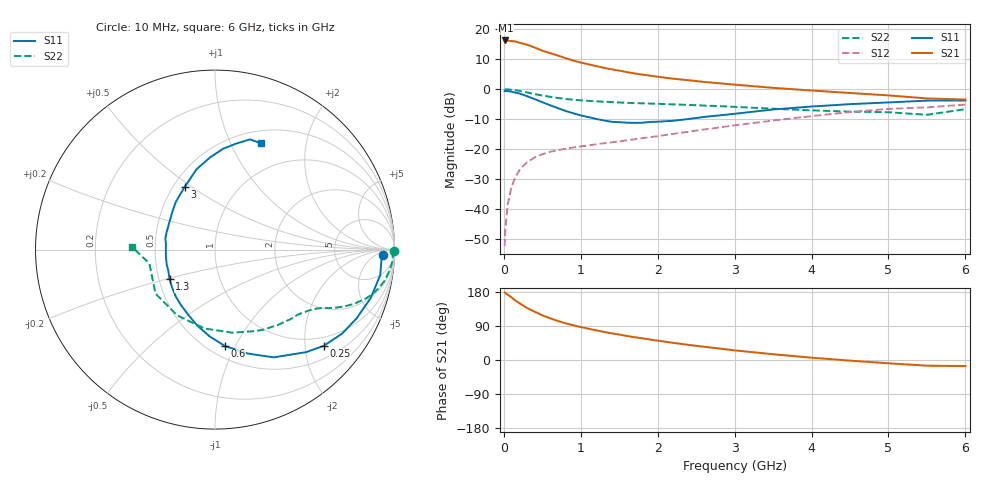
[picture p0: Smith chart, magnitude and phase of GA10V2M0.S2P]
! Infineon Technologies  Discrete & RF Semiconductors
! BF775
! Si NPN RF Bipolar Junction Transistor in SOT23
! VCE = 10 V  IC = 2 mA
! Common Emitter S-Parameters:  May  1996
# GHz  S  MA  R  50
!  f  S11  S21  S12  S22
! GHz  MAG  ANG  MAG  ANG  MAG  ANG  MAG  ANG
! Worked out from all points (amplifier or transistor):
!   36 points, 10 MHz to 6 GHz, reference 50 ohm
!   highest |S21| = 16.3 dB at 20 MHz (marker M1)
!   |S21| within 3 dB of that: start of sweep to 461.3 MHz
!   unconditionally stable (mu >= 1): 1.235 GHz to 3.193 GHz
!   at 250 MHz: K = 0.27, MSG = 20.4 dB, |S12| = -25.7 dB
!   at 1.4 GHz: K = 1.06, MAG = 10.6 dB, |S12| = -17.7 dB
!   at 6 GHz: K = 0.93, MSG = 0.8 dB, |S12| = -5.1 dB
!   S11 on the Smith chart (normalised r, x): 10 MHz: 24, -11; 250 MHz: 0.78, -2.42; 600 MHz: 0.60, -0.91; 1.3 GHz: 0.57, -0.20; 3 GHz: 0.57, +0.47; 6 GHz: 0.65, +1.31
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0.01  0.9347 -1.8  6.429 178.5  0.0024 95.5  0.999 -0.6
0.02  0.9292 -3.4  6.508 176.7  0.0046 85.2  0.9906 -1.4
0.05  0.9316 -8.7  6.477 172.4  0.0119 85.0  0.9916 -3.6
0.1  0.9084 -17.3  6.345 165.2  0.0235 79.9  0.9791 -6.9
0.15  0.877 -25.9  6.27 156.9  0.0339 75.0  0.9615 -10.3
0.25  0.809 -41.5  5.759 143.8  0.0521 67.2  0.9123 -15.7
0.3  0.7641 -48.4  5.544 137.4  0.0602 63.6  0.8842 -17.9
0.4  0.6839 -61.4  4.961 127.5  0.0725 58.4  0.8304 -21.4
0.5  0.6071 -72.5  4.397 117.9  0.082 54.1  0.7848 -23.8
0.6  0.5404 -84.1  4.013 110.1  0.0901 51.5  0.7477 -25.6
0.7  0.4841 -93.6  3.656 103.2  0.0959 49.7  0.7152 -27.1
0.8  0.4344 -103.2  3.306 97.0  0.1011 48.5  0.6884 -28.2
0.9  0.3973 -111.1  3.013 91.8  0.1065 48.1  0.6675 -29.3
1.1  0.3419 -129.4  2.6 82.5  0.1157 47.7  0.6394 -31.5
1.3  0.3012 -147.2  2.278 74.2  0.1251 48.3  0.6179 -33.6
1.7  0.2737 -179.9  1.832 60.2  0.146 50.9  0.5849 -38.5
2.2  0.2971 148.5  1.498 45.3  0.1796 52.4  0.5576 -46.3
3  0.3886 115.6  1.192 25.4  0.2493 51.0  0.5072 -63.5
3.5  0.459 103.0  1.053 15.2  0.2997 47.6  0.4726 -78.3
4.5  0.5632 85.5  0.864 -1.7  0.4151 36.7  0.4226 -119.7
5.5  0.6443 72.4  0.701 -15.0  0.4977 20.0  0.3737 -168.1
6  0.6459 66.5  0.671 -16.1  0.5538 15.3  0.4643 178.0
